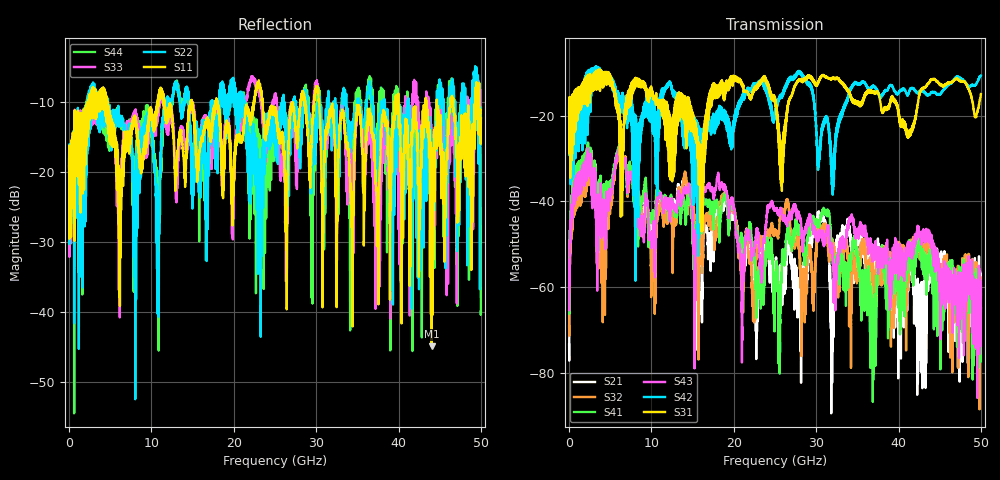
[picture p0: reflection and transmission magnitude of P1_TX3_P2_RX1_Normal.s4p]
!Keysight Technologies,N5225B,MY57041031,A.13.20.10
!Date: Friday, May 31, 2019 11:28:18
!Correction: S11(Full 4 Port(1,2,3,4))
!S12(Full 4 Port(1,2,3,4))
!S13(Full 4 Port(1,2,3,4))
!S14(Full 4 Port(1,2,3,4))
!S21(Full 4 Port(1,2,3,4))
!S22(Full 4 Port(1,2,3,4))
!S23(Full 4 Port(1,2,3,4))
!S24(Full 4 Port(1,2,3,4))
!S31(Full 4 Port(1,2,3,4))
!S32(Full 4 Port(1,2,3,4))
!S33(Full 4 Port(1,2,3,4))
!S34(Full 4 Port(1,2,3,4))
!S41(Full 4 Port(1,2,3,4))
!S42(Full 4 Port(1,2,3,4))
!S43(Full 4 Port(1,2,3,4))
!S44(Full 4 Port(1,2,3,4))
!S4P File: Measurements: <S11,S12,S13,S14>,
!<S21,S22,S23,S24>,
!<S31,S32,S33,S34>,
!<S41,S42,S43,S44>:
# Hz S  dB  R 50.0
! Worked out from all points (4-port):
!   5000 points, 10 MHz to 50 GHz, reference 50 ohm
!   strongest paths, dB at 10 MHz, 12.51 GHz, 25.01 GHz, 37.51 GHz, 50 GHz:
!     S31: -19.4, -27.2, -15.7, -14.5, -14.9
!     S42: -19.4, -14.3, -20.1, -14.6, -10.6
!     S43: -65.4, -40.6, -42.0, -51.3, -59.8
!     S41: -63.2, -40.5, -56.6, -54.5, -61.7
!     S32: -69.0, -46.1, -47.1, -52.9, -57.8
!     S21: -73.4, -45.0, -55.0, -51.8, -65.0
!   lowest |S11| = -44.9 dB at 44.03 GHz (marker M1), VSWR 1.01, Z = 49.8 + j0.535 ohm
!   |S11| at or under -10 dB: 4.66 GHz to 10.77 GHz (6.106 GHz wide, 79.2 % of centre); 23.49 GHz to 28.08 GHz (4.582 GHz wide, 17.8 % of centre); 30.38 GHz to 39.49 GHz (9.118 GHz wide, 26.1 % of centre)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
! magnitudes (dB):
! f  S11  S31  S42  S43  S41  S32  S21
! 10 MHz  -19.5  -19.4  -19.4  -65.4  -63.2  -69.0  -73.4
! 820 MHz  -15.6  -16.1  -18.4  -35.3  -32.9  -37.6  -35.1
! 4.24 GHz  -9.8  -11.8  -10.4  -40.1  -36.0  -45.7  -39.8
! 6.18 GHz  -39.1  -29.2  -15.9  -28.1  -27.7  -27.9  -27.3
! 15.54 GHz  -20.2  -24.9  -21.8  -45.2  -45.9  -51.4  -59.9
! 44.03 GHz  -44.9  -11.4  -14.5  -49.9  -53.2  -53.1  -54.8
! 50 GHz  -12.4  -14.9  -10.6  -59.8  -61.7  -57.8  -65.0
